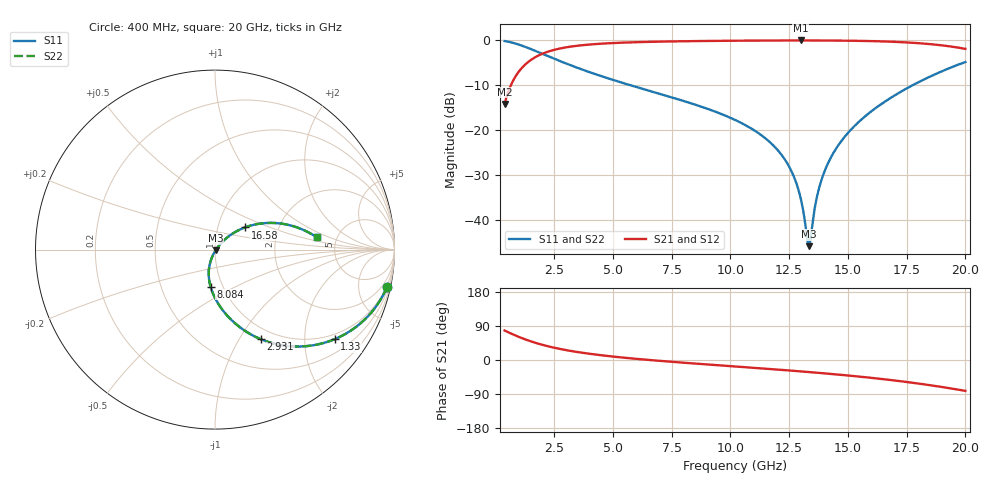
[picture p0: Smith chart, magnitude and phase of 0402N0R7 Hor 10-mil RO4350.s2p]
# GHz S MA R 50
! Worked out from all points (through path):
!   1960 points, 400 MHz to 20 GHz, reference 50 ohm
!   highest |S21| = -0.05 dB at 13 GHz (marker M1); lowest = -14.2 dB at 400 MHz (marker M2)
!   lowest |S11| = -45.9 dB at 13.34 GHz (marker M3), VSWR 1.01, Z = 50.4 - j0.296 ohm
!   |S11| at or under -10 dB: 5.736 GHz to 17.76 GHz (12.03 GHz wide, 102 % of centre)
!   |S22| runs from -45.9 to -0.2 dB; largest |S21 - S12| = 0
!   S11 on the Smith chart (normalised r, x): 400 MHz: 0.85, -9.25; 1.33 GHz: 0.85, -2.78; 2.931 GHz: 0.85, -1.25; 8.084 GHz: 0.88, -0.38; 16.58 GHz: 1.35, +0.35; 20 GHz: 3.52, +0.71
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0.4  0.9807 -12.2  0.1953 77.8  0.1953 77.8  0.9807 -12.2
0.8102093  0.9273 -23.9  0.3741 66.0  0.3741 66.0  0.9273 -23.9
1.330475  0.8332 -36.8  0.5524 53.2  0.5524 53.2  0.8332 -36.8
2.931291  0.5619 -62.8  0.826 27.1  0.826 27.1  0.5619 -62.8
3.671669  0.4746 -70.4  0.8788 19.4  0.8788 19.4  0.4746 -70.4
6.943338  0.2554 -91.5  0.9644 -2.0  0.9644 -2.0  0.2554 -91.5
8.08392  0.2079 -96.8  0.9754 -7.5  0.9754 -7.5  0.2079 -96.8
10.205  0.1294 -105.6  0.9879 -17.1  0.9879 -17.1  0.1294 -105.6
12.07596  0.05724 -111.4  0.9937 -25.6  0.9937 -25.6  0.05724 -111.4
12.62624  0.03371 -110.5  0.9944 -28.2  0.9944 -28.2  0.03371 -110.5
12.99643  0.01723 -103.8  0.9945 -30.0  0.9945 -30.0  0.01723 -103.8
13.26656  0.006245 -67.9  0.9944 -31.4  0.9944 -31.4  0.006245 -67.9
13.3366  0.005083 -35.2  0.9944 -31.7  0.9944 -31.7  0.005083 -35.2
13.46667  0.008005 17.3  0.9942 -32.4  0.9942 -32.4  0.008005 17.3
13.62675  0.01513 36.2  0.994 -33.2  0.994 -33.2  0.01513 36.2
13.80684  0.0241 42.7  0.9937 -34.2  0.9937 -34.2  0.0241 42.7
14.36713  0.05446 46.5  0.9919 -37.2  0.9919 -37.2  0.05446 46.5
15.26759  0.1098 43.9  0.9863 -42.4  0.9863 -42.4  0.1098 43.9
16.57825  0.2074 36.5  0.9687 -51.0  0.9687 -51.0  0.2074 36.5
16.73834  0.2209 35.4  0.9655 -52.2  0.9655 -52.2  0.2209 35.4
18.53925  0.3985 21.3  0.9034 -66.9  0.9034 -66.9  0.3985 21.3
20  0.5718 6.8  0.8019 -81.4  0.8019 -81.4  0.5718 6.8
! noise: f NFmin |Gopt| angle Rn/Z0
0.4  0.001326  0.8422  6.649  0.001776
2.571  0.004587  0.6585  10.31  0.002545
4.752  0.007417  0.6148  14.4  0.003527
6.933  0.01025  0.5979  18.83  0.004574
9.104  0.01334  0.5968  23.27  0.005851
11.29  0.01699  0.6081  27.68  0.007595
13.47  0.02158  0.631  32.02  0.01019
15.64  0.02776  0.6648  36.3  0.0144
17.82  0.03695  0.7104  40.63  0.02218
20  0.05233  0.7679  45.08  0.03926
